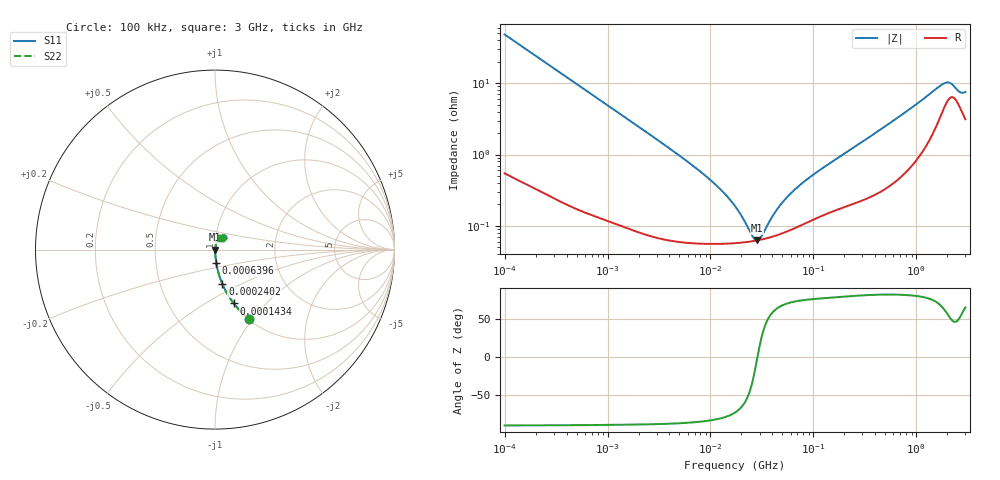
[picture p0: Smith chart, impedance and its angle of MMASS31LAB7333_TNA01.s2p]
! MMASS31LAB7333_TNA01  S-PARAMETER MODEL  ( Standard Model )
! Model Generated by TAIYO YUDEN Corporation (http://www.ty-top.com)
! Version 1.0
! TAIYO YUDEN Control No. 220601
! Copyright(c) 2018 TAIYO YUDEN CO.,LTD. All Rights Reserved.
! Product Description (link to TY-COMPAS)
! https://ds.yuden.co.jp/TYCOMPAS/or/detail?pn=MMASS31LAB7333KTNA01&u=M
! Products Name : Multilayer Ceramic Capacitors
! Characteristics :
!  Capacitance : 0.033 [uF] , Rated Voltage : 630 [V] , TCC : X7R
!  Case Size : 3.2 x 1.6 / 0.126 x 0.063 [mm/inch] , Thickness : 1.6 / 0.063 [mm/inch]
!  (Conditions: Temperature = 25 [degC] , DC Bias Voltage = 0 [V])
! External Node Assignments :
!  1  o---| |---o  2
! GND o---------o GND
! Frequency Range : 100kHz  -  3GHz  [ 401 STEP ]
# MHZ S RI R 50
! Freq[MHz].  S11 Real  S11 Imag  S21 Real  S21 Imag  S12 Real  S12 Imag  S22 Real  S22 Imag
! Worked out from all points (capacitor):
!   401 points, 100 kHz to 3 GHz, reference 50 ohm
!   read as one part in series: C = 33 nF near 105.3 kHz
!   lowest |Z| = 62.7 mohm at 28.26 MHz (marker M1)
!   series resonance near 28.59 MHz, so ESL is about 940 pH
!   S11 on the Smith chart (normalised r, x): 100 kHz: 1.01, -0.96; 143.4 kHz: 1.01, -0.67; 240.2 kHz: 1.01, -0.40; 639.6 kHz: 1.00, -0.15; 3 GHz: 1.06, +0.14
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0.1  0.1912 -0.3876  0.8088 0.3876  0.8088 0.3876  0.1912 -0.3876
0.14345  0.1048 -0.3002  0.8952 0.3002  0.8952 0.3002  0.1048 -0.3002
0.24019  0.0417 -0.1929  0.9583 0.1929  0.9583 0.1929  0.0417 -0.1929
0.562235  0.00904 -0.0859  0.991 0.0859  0.991 0.0859  0.00904 -0.0859
0.639561  0.00726 -0.0757  0.9927 0.0757  0.9927 0.0757  0.00726 -0.0757
3.161081  0.000908 -0.0155  0.9991 0.0155  0.9991 0.0155  0.000908 -0.0155
9.824692  0.000579 -0.00445  0.9994 0.00445  0.9994 0.00445  0.000579 -0.00445
13.7349  0.00057 -0.00278  0.9994 0.00278  0.9994 0.00278  0.00057 -0.00278
17.7727  0.000577 -0.00171  0.9994 0.00171  0.9994 0.00171  0.000577 -0.00171
25.49486  0.000609 -0.000395  0.9994 0.000395  0.9994 0.000395  0.000609 -0.000395
28.26337  0.000625 -3.94e-05  0.9994 3.94e-05  0.9994 3.94e-05  0.000625 -3.94e-05
31.3325  0.000644 0.000314  0.9994 -0.000314  0.9994 -0.000314  0.000644 0.000314
40.54368  0.000711 0.00121  0.9993 -0.00121  0.9993 -0.00121  0.000711 0.00121
51.12795  0.000801 0.00206  0.9992 -0.00206  0.9992 -0.00206  0.000801 0.00206
67.88584  0.000956 0.00321  0.999 -0.00321  0.999 -0.00321  0.000956 0.00321
97.38194  0.00123 0.00494  0.9988 -0.00494  0.9988 -0.00494  0.00123 0.00494
547.5153  0.00431 0.0269  0.9957 -0.0269  0.9957 -0.0269  0.00431 0.0269
1217.231  0.0159 0.0599  0.9841 -0.0599  0.9841 -0.0599  0.0159 0.0599
1838.476  0.0482 0.0809  0.9518 -0.0809  0.9518 -0.0809  0.0482 0.0809
2091.327  0.0629 0.0721  0.9371 -0.0721  0.9371 -0.0721  0.0629 0.0721
2637.286  0.0475 0.054  0.9525 -0.054  0.9525 -0.054  0.0475 0.054
3000  0.0345 0.0645  0.9655 -0.0645  0.9655 -0.0645  0.0345 0.0645
